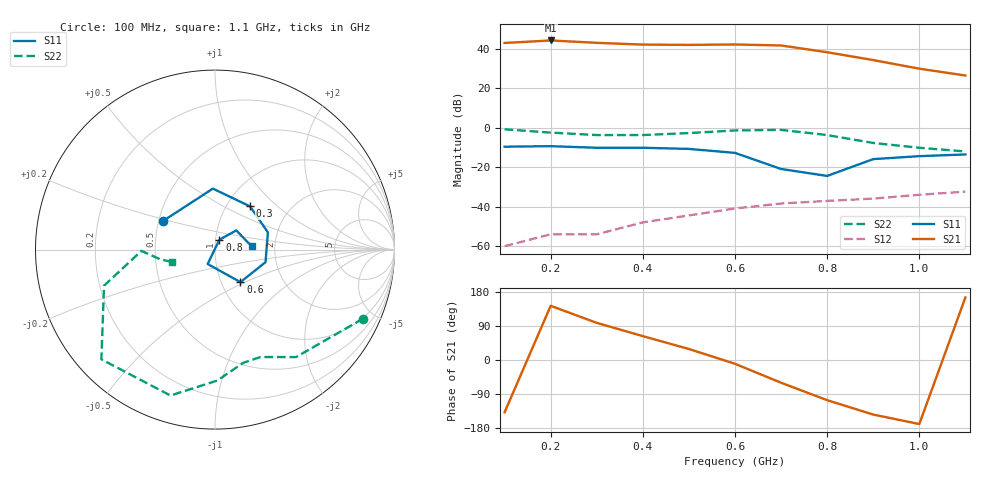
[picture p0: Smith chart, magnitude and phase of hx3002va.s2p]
!  HPMX-3002  S PARAMETERS
!  Vcc1=4.5 V, Vcc2=6 V, Vcontrol = 1.6 V
!  LAST UPDATED 01 07 94
# ghz s ma r 50
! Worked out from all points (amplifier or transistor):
!   11 points, 100 MHz to 1.1 GHz, reference 50 ohm
!   highest |S21| = 44.2 dB at 200 MHz (marker M1)
!   |S21| within 3 dB of that: start of sweep to 713.4 MHz
!   unconditionally stable (mu >= 1): 262.9 MHz to 321.5 MHz; 964.5 MHz to end of sweep
!   at 200 MHz: K = 0.82, MSG = 49.1 dB, |S12| = -54.0 dB
!   at 600 MHz: K = 0.62, MSG = 41.5 dB, |S12| = -40.9 dB
!   at 1.1 GHz: K = 1.14, MAG = 27.1 dB, |S12| = -32.4 dB
!   S11 on the Smith chart (normalised r, x): 100 MHz: 0.53, +0.19; 300 MHz: 1.28, +0.68; 600 MHz: 1.23, -0.47; 800 MHz: 1.04, +0.11; 1.1 GHz: 1.53, +0.07
0.1  0.33 151.0  139.4 -138.0  0.001 143.0  0.91 -25.0
0.2  0.34 92.0  161.4 143.0  0.002 152.0  0.75 -53.0
0.3  0.31 51.0  140.5 98.0  0.002 146.0  0.65 -67.0
0.4  0.31 18.0  126.8 63.0  0.004 148.0  0.65 -76.0
0.5  0.29 -14.0  124.6 29.0  0.006 141.0  0.73 -89.0
0.6  0.23 -52.0  127.7 -10.0  0.009 143.0  0.85 -107.0
0.7  0.09 -117.0  120.5 -60.0  0.012 138.0  0.88 -136.0
0.8  0.06 66.0  81.23 -106.0  0.014 135.0  0.65 -162.0
0.9  0.16 42.0  51.44 -144.0  0.016 131.0  0.41 -179.0
1  0.19 11.0  31.15 -169.0  0.02 130.0  0.31 -170.0
1.1  0.21 6.0  20.93 165.0  0.024 127.0  0.25 -164.0
